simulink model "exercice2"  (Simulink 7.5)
settings: Solver=ode45  StartTime=0.0  StopTime=10.0  RelTol=1e-3

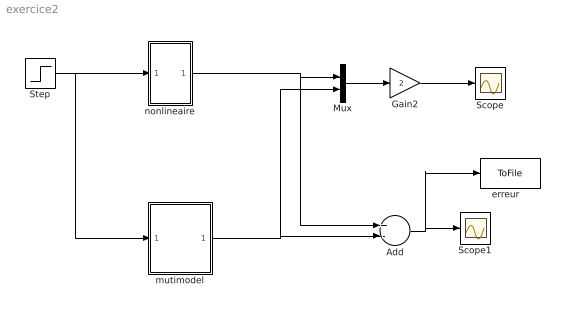
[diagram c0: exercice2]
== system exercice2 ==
  Add : Sum  Inputs=+-  OutDataType=fixdt(1, 16)  OutScaling=2^-10
  Gain2 : Gain  Gain=2  ParameterDataType=fixdt(1, 16)  ParameterScaling=2^0  OutDataType=fixdt(1, 16)  OutScaling=2^0
  Mux : Mux  Inputs=2
  Scope : Scope
  Scope1 : Scope
  Step : Step  SampleTime=0
  "erreur   " : ToFile  Filename=erreur
  mutimodel : Subsystem
  nonlineaire : Subsystem
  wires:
  Gain2/1 -> Scope/1
  Step/1 -> nonlineaire/1(In1), mutimodel/1(In1)
  Mux/1 -> Gain2/1
  mutimodel/1(u) -> Mux/2, Add/2
  nonlineaire/1(Out1) -> Mux/1, Add/1
  Add/1 -> Scope1/1, "erreur   "/1

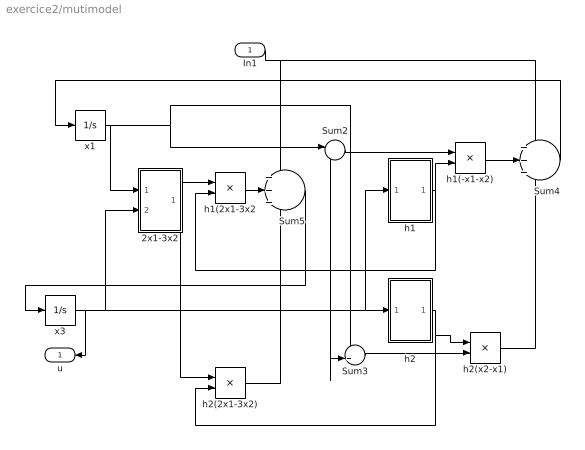
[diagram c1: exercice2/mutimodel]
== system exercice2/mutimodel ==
  In1 : Inport
  2x1-3x2 : Subsystem
  Sum2 : Sum  Inputs=--  OutDataType=fixdt(1, 16)  OutScaling=2^0
  Sum3 : Sum  Inputs=-+  OutDataType=fixdt(1, 16)  OutScaling=2^0
  Sum4 : Sum  Inputs=+++  OutDataType=fixdt(1, 16)  OutScaling=2^0
  Sum5 : Sum  Inputs=+++  OutDataType=fixdt(1, 16)  OutScaling=2^0
  h1 : Subsystem
  h1(-x1-x2) : Product  OutDataType=fixdt(1, 16)  OutScaling=2^0
  h1(2x1-3x2 : Product  OutDataType=fixdt(1, 16)  OutScaling=2^0
  h2 : Subsystem
  h2(2x1-3x2) : Product  OutDataType=fixdt(1, 16)  OutScaling=2^0
  h2(x2-x1) : Product  OutDataType=fixdt(1, 16)  OutScaling=2^0
  x1 : Integrator
  x3 : Integrator
  u : Outport
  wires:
  x3/1 -> h2/1(In1), h1/1(In1), Sum2/2, Sum3/2, 2x1-3x2/2(In2), u/1
  x1/1 -> Sum2/1, Sum3/1, 2x1-3x2/1(In1)
  Sum2/1 -> h1(-x1-x2)/1
  h1/1(Out1) -> h1(-x1-x2)/2, h1(2x1-3x2/2
  Sum3/1 -> h2(x2-x1)/2
  h2/1(Out1) -> h2(x2-x1)/1, h2(2x1-3x2)/2
  h1(-x1-x2)/1 -> Sum4/2
  h2(x2-x1)/1 -> Sum4/3
  Sum4/1 -> x1/1
  2x1-3x2/1(Out1) -> h1(2x1-3x2/1, h2(2x1-3x2)/1
  h2(2x1-3x2)/1 -> Sum5/3
  h1(2x1-3x2/1 -> Sum5/2
  Sum5/1 -> x3/1
  In1/1 -> Sum4/1, Sum5/1

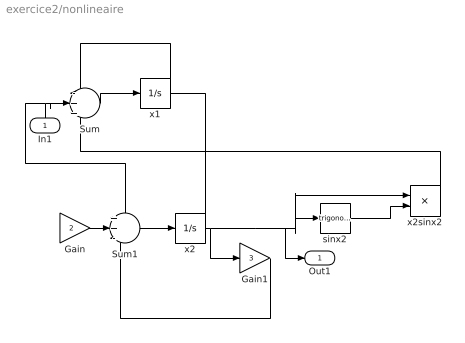
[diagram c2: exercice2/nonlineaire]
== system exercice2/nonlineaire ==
  In1 : Inport
  Gain : Gain  Gain=2  ParameterDataType=fixdt(1, 16)  ParameterScaling=2^0  OutDataType=fixdt(1, 16)  OutScaling=2^0
  Gain1 : Gain  Gain=3  ParameterDataType=fixdt(1, 16)  ParameterScaling=2^0  OutDataType=fixdt(1, 16)  OutScaling=2^0
  Sum : Sum  Inputs=-++  OutDataType=fixdt(1, 16)  OutScaling=2^0
  Sum1 : Sum  Inputs=++-  OutDataType=fixdt(1, 16)  OutScaling=2^0
  sinx2 : Trigonometry
  x1 : Integrator
  x2 : Integrator
  x2sinx2 : Product  OutDataType=fixdt(1, 16)  OutScaling=2^0
  Out1 : Outport
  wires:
  Sum/1 -> x1/1
  x1/1 -> Sum/1, Gain/1
  In1/1 -> Sum1/1, Sum/2
  Gain/1 -> Sum1/2
  Sum1/1 -> x2/1
  Gain1/1 -> Sum1/3
  x2/1 -> Gain1/1, x2sinx2/1, sinx2/1, Out1/1
  sinx2/1 -> x2sinx2/2
  x2sinx2/1 -> Sum/3

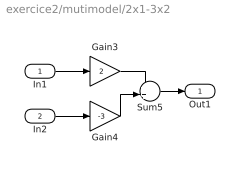
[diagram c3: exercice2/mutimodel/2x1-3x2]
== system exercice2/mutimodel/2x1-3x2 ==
  In1 : Inport
  In2 : Inport  Port=2
  Gain3 : Gain  Gain=2  ParameterDataType=fixdt(1, 16)  ParameterScaling=2^0  OutDataType=fixdt(1, 16)  OutScaling=2^0
  Gain4 : Gain  Gain=-3  ParameterDataType=fixdt(1, 16)  ParameterScaling=2^0  OutDataType=fixdt(1, 16)  OutScaling=2^0
  Sum5 : Sum  OutDataType=fixdt(1, 16)  OutScaling=2^0
  Out1 : Outport
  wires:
  Gain3/1 -> Sum5/1
  Gain4/1 -> Sum5/2
  In1/1 -> Gain3/1
  In2/1 -> Gain4/1
  Sum5/1 -> Out1/1

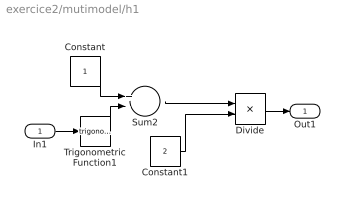
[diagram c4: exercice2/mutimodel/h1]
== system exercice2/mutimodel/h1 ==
  In1 : Inport
  Constant : Constant  OutDataType=fixdt(1, 16)  OutScaling=2^0
  Constant1 : Constant  Value=2  OutDataType=fixdt(1, 16)  OutScaling=2^0
  Divide : Product  Inputs=*/  OutDataType=fixdt(1, 16)  OutScaling=2^-10
  Sum2 : Sum  Inputs=+-  OutDataType=fixdt(1, 16)  OutScaling=2^0
  Trigonometric Function1 : Trigonometry
  Out1 : Outport
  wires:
  Constant/1 -> Sum2/1
  Trigonometric Function1/1 -> Sum2/2
  Sum2/1 -> Divide/1
  Constant1/1 -> Divide/2
  Divide/1 -> Out1/1
  In1/1 -> Trigonometric Function1/1

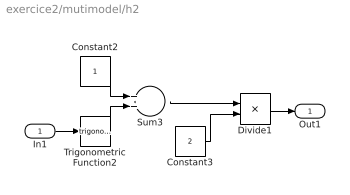
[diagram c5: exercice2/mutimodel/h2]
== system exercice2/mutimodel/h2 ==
  In1 : Inport
  Constant2 : Constant  OutDataType=fixdt(1, 16)  OutScaling=2^0
  Constant3 : Constant  Value=2  OutDataType=fixdt(1, 16)  OutScaling=2^0
  Divide1 : Product  Inputs=*/  OutDataType=fixdt(1, 16)  OutScaling=2^-10
  Sum3 : Sum  OutDataType=fixdt(1, 16)  OutScaling=2^0
  Trigonometric Function2 : Trigonometry
  Out1 : Outport
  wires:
  Constant2/1 -> Sum3/1
  Trigonometric Function2/1 -> Sum3/2
  Sum3/1 -> Divide1/1
  Constant3/1 -> Divide1/2
  Divide1/1 -> Out1/1
  In1/1 -> Trigonometric Function2/1
